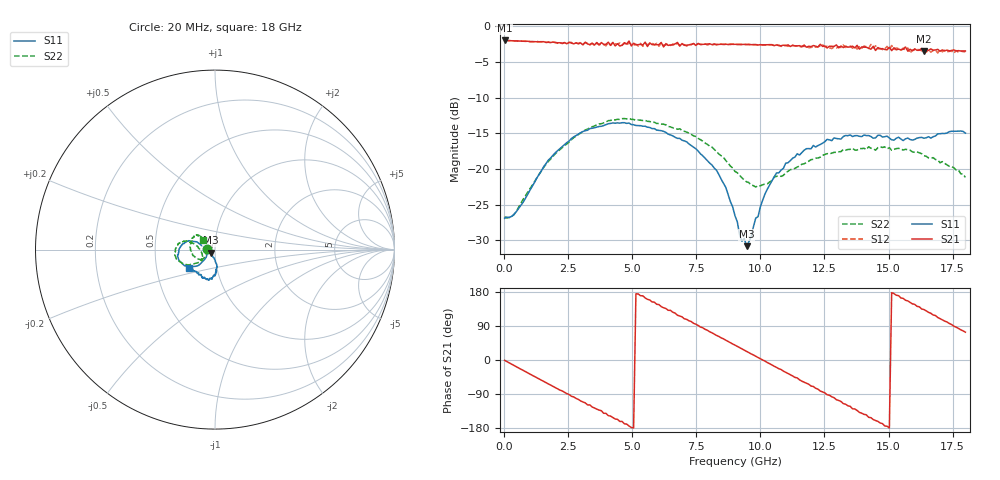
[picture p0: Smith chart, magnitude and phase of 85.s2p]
!Agilent Technologies,N5230A,US43500223,A.07.50.48
!Agilent N5230A: A.07.50.48
!Date: Monday, January 18, 2016 14:53:15
!Correction: S11(Full 2 Port(1,2))
!S21(Full 2 Port(1,2))
!S12(Full 2 Port(1,2))
!S22(Full 2 Port(1,2))
!S2P File: Measurements: S11, S21, S12, S22:
# Hz S  dB  R 50
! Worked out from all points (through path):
!   201 points, 20 MHz to 18 GHz, reference 50 ohm
!   highest |S21| = -1.97 dB at 20 MHz (marker M1); lowest = -3.5 dB at 16.38 GHz (marker M2)
!   group delay of S21, straight-line fit = 99.6 ps
!   lowest |S11| = -30.8 dB at 9.46 GHz (marker M3), VSWR 1.06, Z = 47.7 - j1.61 ohm
!   |S11| at or under -10 dB: start of sweep to end of sweep
!   |S22| runs from -26.9 to -12.9 dB; largest |S21 - S12| = 0.073
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2e7  -26.89 179.2  -1.97 -0.8  -1.97 -0.9  -26.67 179.0
8.291e8  -24.12 -140.7  -2.09 -30.5  -2.09 -30.6  -23.78 -146.5
1.5483e9  -19.65 -135.5  -2.15 -56.7  -2.13 -57.1  -19.74 -140.6
2.5372e9  -16.08 -143.0  -2.23 -91.1  -2.24 -91.0  -16.24 -147.7
3.0766e9  -14.73 -149.2  -2.59 -110.9  -2.49 -111.3  -14.74 -153.0
3.7958e9  -14.00 -158.2  -2.26 -133.9  -2.51 -134.4  -13.64 -161.7
4.8746e9  -13.54 -172.1  -2.04 -174.3  -2.26 -173.4  -12.86 -175.0
6.0433e9  -14.57 171.7  -2.56 146.2  -2.78 144.6  -13.61 172.3
6.7625e9  -15.70 163.8  -2.25 118.1  -2.34 118.1  -14.42 166.8
7.5716e9  -17.46 159.8  -2.39 91.3  -2.42 90.7  -15.69 162.9
8.2908e9  -20.18 158.8  -2.58 64.8  -2.52 64.0  -17.54 163.7
9.01e9  -26.55 177.8  -2.51 39.3  -2.55 37.9  -20.34 170.6
9.4595e9  -30.80 -144.1  -2.53 22.7  -2.55 21.8  -21.79 -178.2
1.06282e10  -20.55 -82.8  -2.58 -19.4  -2.64 -20.6  -21.02 -145.1
1.20666e10  -16.69 -90.2  -2.68 -69.9  -2.79 -73.0  -18.64 -158.3
1.32353e10  -15.43 -101.4  -2.97 -115.1  -2.62 -114.6  -17.24 -179.3
1.43141e10  -15.43 -109.0  -3.19 -152.2  -2.53 -155.4  -17.08 162.0
1.50333e10  -15.65 -117.5  -2.94 -179.5  -3.30 -179.8  -16.99 151.3
1.57525e10  -15.65 -127.1  -3.46 156.0  -3.03 153.1  -17.28 144.0
1.63818e10  -15.67 -133.3  -3.48 133.0  -3.14 128.3  -18.13 141.4
1.69212e10  -15.06 -140.0  -3.21 112.1  -3.73 110.9  -18.73 137.7
1.8e10  -14.95 -145.5  -3.44 73.5  -3.56 71.1  -21.16 140.6
